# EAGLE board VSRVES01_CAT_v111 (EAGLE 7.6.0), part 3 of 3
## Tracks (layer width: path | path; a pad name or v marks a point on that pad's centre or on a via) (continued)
HP_LEFT  (via drill 0.4) (continued)
  Top 0.3: 3.3,41.7 4.2,42.6 4.2,45 6.2,47 6.4,47.2 HP-OUT.4 | R29.2 10.25,48.15
  Bottom 0.2: 7.4,48.2 HP-OUT.4
  Bottom 0.3: v10.2,48.2 7.4,48.2 HP-OUT.4
HP_MUTE  (via drill 0.4)
  Top 0.2: U4.4 3.2,40.4 5,38.6 v5,38.2 | v3.2,37.6 3.2,35.8 4,35 4.15,35 R37.1
  Bottom 0.2: v5,38.2 3.8,38.2 v3.2,37.6
HP_RIGHT
  Top 0.2: U4.13 9.1,41.7 9.2,41.8
  Top 0.3: 9.2,41.8 9.2,45 8.6,45.6 8.6,46.4 9.2,47 9.2,52.1 HP-OUT.1 9.9,52.75 R27.2
INT_N
  Top 0.2: U2.38 44.2,66.38 44.2,67 43.8,67.4 43.8,68 43.8,68.4 44,68.6 R7.1
LINE_ADC_L  (via drill 0.3)
  Top 0.2: U1.81 v17.4,39.02 | v8.6,55.4 6.6,55.4 5.8,56.2 R24.2 5.78,57.33 C25.1
  Bottom 0.2: v17.4,39.02 17.4,40.4 16.4,41.4 16.4,46.8 15.6,47.6 15.6,52.4 12.6,55.4 v8.6,55.4
LINE_ADC_R  (via drill 0.3)
  Top 0.2: U1.80 18,38.99 v18,39.49 | v11.4,56.2 11.2,56.4 R25.2 9.43,57.35 C27.1
  Bottom 0.2: v18,39.49 18,40.4 16.8,41.6 16.8,47 16,47.8 16,52.6 12.6,56 11.6,56 v11.4,56.2
MCT1  (via drill 0.4)
  Top 0.2: v35.8,67.2 C11.1
  Bottom 0.2: J1.P2 22.64,72.4 30,72.4 31,71.4 31,68.4 32.2,67.2 v35.8,67.2
MCT2  (via drill 0.4)
  Top 0.2: C10.1 v34.2,66.4
  Bottom 0.2: J1.P5 27.07,66.4 v34.2,66.4
MDC  (via drill 0.3)
  Top 0.2: U1.59 29.2,40.78 29.2,44.6 30.8,46.2 35.4,46.2 35.8,45.8 45.6,45.8 v46.4,46.6 | U2.36 46.4,66.09 46.4,67 47.2,67.8 v47.6,67.8 R9.1
  Bottom 0.2: v46.4,46.6 49.4,49.6 51.4,49.6 51.6,49.8 51.6,57.4 53.6,59.4 53.6,64.6 52.6,65.6 49.4,65.6 47.6,67.4 v47.6,67.8 47,67.8 46.6,67.4 45.6,67.4 45,68 45,75.4 44.13,76.27 JP3.2
MDIO  (via drill 0.3)
  Top 0.2: U1.58 29.6,40.61 29.6,44.4 31,45.8 35.2,45.8 35.8,45.2 46,45.2 v46.8,46 | U2.37 44.8,66.49 44.8,67.2 45.6,68 v45.8,68 R8.1
  Bottom 0.2: v46.8,46 50,49.2 51.8,49.2 52,49.4 52,57.2 54,59.2 54,65 53,66 49.6,66 48.2,67.4 48.2,68.2 47.8,68.6 46.6,68.6 46,68 v45.8,68 45.8,80.8 46.67,81.67 JP3.3
MX1+  (via drill 0.3)
  Top 0.2: U2.2 41.22,60.2 34.2,60.2 33.8,60.6 v33,60.6
  Bottom 0.2: J1.P1 19.95,67.25 22.2,65 30.6,65 33,62.6 v33,60.6
MX1-  (via drill 0.3)
  Top 0.2: U2.3 41.52,59.8 v33.6,59.8
  Bottom 0.2: J1.P3 22.5,66.91 23.8,65.6 31,65.6 33.6,63 v33.6,59.8
MX2+
  Top 0.2: U2.5 40.94,57.8 34.6,57.8 32,60.4 32,64.6 30.2,66.4 30.2,71.6 29.4,72.4 25.18,72.4 J1.P4
MX2-
  Top 0.2: U2.6 41.25,57.4 34.2,57.4 31.4,60.2 31.4,64.4 29.6,66.2 29.6,69 28.8,69.8 27.48,69.8 J1.P6
N$1
  Top 0.2: JMP1.1 14.95,44.8 14.31,44.8 14.01,44.5 U3.4 13.55,43.55 13.2,43.2 12,43.2 11.65,42.85 U3.1
N$2  (via drill 0.4)
  Top 0.2: U2.16 47.39,58.21 48,57.6 48,57 48.2,56.8 | 47.08,55.08 C33.1 | U2.40 43.4,65.77 43.4,66.2 43.14,66.46 41.8,66.46 41.6,66.66 41.6,67 | U2.34 48.92,67.2 | 46.08,55.08 v46.1,55.1
  Top 0.3: 48.2,56.8 48.2,56.2 47.08,55.08 | 48.92,67.2 50.2,67.2 v50.8,67.8 51,68 C16.1 | v46.4,56 46.4,55.6 46.8,55.2 46.88,55.2 C33.1 46.08,55.08 45.8,54.8 45.8,51.6 FB5.2 45.2,51.6 44.2,50.6 44.2,50.2 43.4,49.4 C43.1 | C17.1 41.6,67 v42.2,67
  POW 0.4: v42.2,67 48.4,67 | 48.4,67 48.6,67.2 50.2,67.2 v50.8,67.8 | 48.4,67 48.4,63.2 49.2,62.4 49.2,59.8 46.4,57 v46.4,56 46.4,55.4 v46.1,55.1
  Bottom 0.3: C114.1 v46.4,56 | C121.1 41.8,67 v42.2,67
N$3
  Top 0.2: U7.7 4.12,19.35 C66.2 4.67,18.07 4.4,17.8 1.8,17.8 0.6,19 0.6,25.6 0.95,25.95 R50.2 0.95,28.5 R43.1
N$4
  Top 0.2: C61.2 8.35,26.8 R44.1 | R41.2 6.65,26.82 C61.2 | U7.1 6,25 6.67,25.68 C61.2
N$5  (via drill 0.4)
  Top 0.2: 39.2,60.8 39.4,61.2 | 39.4,61.2 39.2,61.4 | U2.12 44.8,56.71 C32.1 | U2.1 40.91,60.6 40,60.6 39.8,60.8 39.4,60.8 39.4,61.2
  Top 0.3: C22.1 39.2,61.4 | 41.48,53 C37.1 | 44.73,55 C32.1
  Top 0.4: 39.2,61.4 v40,61.4 | FB4.2 39.8,52.8 41.48,52.8 41.48,53 | C37.1 C38.1 43.2,54.4 v43.8,55 44.73,55
  Bottom 0.3: C117.1 39.2,61.4 v40,61.4
  Bottom 0.4: v43.8,55 43.8,57.6 v40,61.4
N$6  (via drill 0.3)
  Top 0.2: RE.C 44.6,42.4 44.4,42.2 42.4,42.2 42.2,42.4 v41.2,42.4
  Bottom 0.2: v41.2,42.4 42.4,41.2 R3.2
N$7  (via drill 0.3)
  Top 0.2: LE.C v39.4,42.2
  Bottom 0.2: v39.4,42.2 40.2,41.4 R4.2
N$8  (via drill 0.4)
  Top 0.2: U2.9 41.57,55.6 | U2.4 41.03,58.6
  Top 0.3: 41.57,55.6 v40,55.6 C30.1
  Top 0.4: 41.03,58.6 v40,58.6 39.8,58.8 C24.1 | FB3.2 37.4,53 37.3,53 v37.3,54
  Bottom 0.3: C116.1 39.2,57.8 | C115.1 39.4,56.2 v40,55.6
  Bottom 0.4: 39.2,57.8 v40,58.6 | v37.3,54 38.4,54 38.5,54.1 39.08,54.67 C115.1 C116.1
N$9  (via drill 0.4)
  Top 0.2: U2.44 42.03,64.31 | 42.03,64.31 41.14,65.2 38.2,65.2 37.4,66 v37.4,67.8 | v37.4,67.8 37.4,68.2 | 37.4,68.2 C12.1 | 37.4,68.2 v37.4,67.8 | 42.03,64.31 42.03,64.57 v42,64.6 | v36.4,72.4 C9.1 37.2,72.53 FB2.2
  Bottom 0.2: v37.4,67.8 37.2,67.8 36.4,68.6 v36.4,72.4
  Bottom 0.3: C119.1 42.4,64.2 v42,64.6
N$11
  Top 0.2: U5.2 11.47,62.08 11.8,62.4 11.93,62.4 C21.1 | C21.1 14.07,62.67 14.2,62.8 13.95,62.8 R21.1 | R16.2 C21.1
N$12
  Top 0.2: R26.1 13.05,57.4 13.8,57.4 15,58.6 15,64 14.6,64.4 R16.1 13.85,65.75 13.4,66.2 XC2.+
N$13
  Top 0.2: R23.1 1.25,58.15 0.4,59 0.4,65.85 R14.1 4.6,70.05 4.6,75 12,82.4 XC1.+
N$14
  Top 0.2: R11.2 3.4,66.85 3.4,67.6 4.6,68.8 5.4,68.8 ADC_JACK.4 8.8,72.2 8.8,76.2 9.6,77 11,77 11.8,76.2 TV2.1 12.9,76.2 12.9,79.2 XC1.-
N$15  (via drill 0.4)
  Top 0.2: C35.1 50.27,55.08 C34.1 48.67,54.88 | U2.18 49.2,57.85 | 47.6,52 47.6,51.88 C39.1 | 47.33,48.52 FB6.2 | U2.39 43.8,66.08 43.8,66.4 | U2.30 49.55,65 | U2.26 50.58,63.2 v51,63.2 | U2.23 50.98,59.6
  Top 0.3: 49.2,57.85 49.2,56.8 49,56.6 C34.1 | 48.67,54.88 v48,54.2 48,52.4 47.6,52 | C39.1 C40.1 47.33,48.52 | 43.8,66.4 42.4,67.8 v42.4,68 42.2,68.2 C15.1 C14.1 C13.1 | 49.55,65 v50.6,65 53,67.4 C19.1 | 50.27,55.08 v49.8,55 | 50.98,59.6 51.52,59.06 53.14,59.06 53.26,59.26
  Top 0.4: v52.4,59.8 52.73,59.8 53.26,59.26 C23.1
  POW 0.4: v49.8,55 48.8,55 | 48.8,55 48.8,56.4 51.6,59.2 51.8,59.2 v52.4,59.8 | 48.8,55 v48,54.2
  Bottom 0.3: 49.67,64.47 C120.1 49.6,64.47 49.6,64.6
  Bottom 0.4: v52.4,59.8 51.8,60.4 51,60.4 49.67,61.73 C118.1 | 49.6,64.6 47.2,67 44.6,67 43.6,68 v42.4,68 | 49.8,64.4 C120.1 C118.1 | 49.6,64.47 49.88,64.47 50.4,65 v50.6,65 | C118.1 49.8,62.8 50.2,63.2 v51,63.2
N$16
  cutout GND: 20.92,84.58 20.92,82.08 26.92,82.08 26.92,84.58
  cutout POW: 20.92,84.58 20.92,82.08 26.92,82.08 26.92,84.58
N$17
  Top 0.2: PWR.C 58.6,1 58,0.4 56.05,0.4 R64.2
N$18
  Top 0.2: R12.2 R15.1
N$19  (via drill 0.3)
  Top 0.2: USD.12 58.95,32.55 v59,32.6
N$20
  Top 0.2: R5.2 10.25,69.85 11.6,71.2 XC2.- 12.9,71.2 12.9,73.6 TV1.1 11,73.6 10.1,74.5 ADC_JACK.1
N$21
  Bottom 0.2: R65.1 55,36.4 53.8,37.6 49.6,37.6 48.65,36.65 U11.4
N$22
  Bottom 0.2: Q1.1 53.15,23.6 C7.1 54.92,25.15 R65.2
N$23  (via drill 0.4)
  Top 0.2: C60.1 52.2,26.4
  Top 0.3: 53.7,27.85 53.85,27.85
  Top 0.4: USD.4 53.85,27.85 | 52.2,26.4 v52.2,27.3 | C60.1 53.7,27.85
  Bottom 0.2: R67.1 52.2,28.4 v52.2,27.3
  Bottom 0.4: Q1.3 v52.2,27.3
N$24  (via drill 0.3)
  Top 0.2: SDPW.A v53.2,33
  Bottom 0.2: R67.2 54,28.4 54,32.2 v53.2,33
N$27
  Top 0.2: R40.2 R41.1 4.92,28.38 C61.1 4.12,26 U7.2
N$30
  Top 0.2: U7.6 3.48,19.35 C66.1 1.8,18.8 1.2,19.4 1.2,25.4 2.6,26.8 R50.1 2.65,28.5 R52.2
N$45
  Top 0.2: R24.1 5.8,59.4 4.8,60.4 3,60.4 2.4,59.8 1.6,59.8 | 1.6,59.8 1.45,59.8 R23.2 | 1.6,59.8 1.6,61.35 | 1.6,61.35 R19.2 | 1.6,61.35 1.77,61.52 C20.2 2.92,61.6 2.8,61.6 3.6,61.6 4.08,62.08 U5.7
N$46
  Top 0.2: R25.1 R26.2 13.65,59.05 14,59.4 14,60.75 R21.2 12.22,60.95 C21.2 11.28,60.92 10.8,61.4 9.82,61.4 U5.1
N$48
  Top 0.2: 1.4,65.2 R14.2 R19.1 2.98,63.25 C20.1 3.12,63.4 3.6,63.4 4.28,62.73 U5.6
N$55
  Top 0.2: JP1.2 R63.2
N$75  (via drill 0.3)
  Top 0.2: RP4.6 52.4,48.8 51,50.2 v51,50.4 | U2.17 48.6,57.74 v48.6,57.4 | R1.2 18.8,57.6 19.2,57.2 24.4,57.2 25.6,58.4 25.6,59.4 26.8,60.6 29.4,60.6 33.8,56.2 34.8,56.2 35.2,55.8 35.2,55 35.6,54.6 41,54.6 41.4,54.2 v42.2,54.2
  Bottom 0.2: v51,50.4 49.8,51.6 49.8,53.4 48.6,54.6 v48.6,57.4 45.8,57.4 45.2,56.8 45.2,55.2 44.2,54.2 v42.2,54.2
N$77  (via drill 0.3)
  Top 0.2: RP4.4 52.6,48 v50.2,50.4 | U2.15 47.6,57.33 v47.6,56.6 | R2.2 24.35,58.55 24.8,59 24.8,60.2 25.8,61.2 29.6,61.2 v34,56.8
  Bottom 0.2: v50.2,50.4 48.2,52.4 47.6,52.4 | 47.6,52.4 46.8,51.6 43.2,51.6 42.4,52.4 36.8,52.4 34,55.2 v34,56.8 | v47.6,56.6 47.2,56.2 47.2,54 47.6,53.6 47.6,52.4
N$78  (via drill 0.3)
  Top 0.2: RP3.2 52,51.2 51.2,52 v50.8,52 | RP2.2 v53,55.2 | U2.19 49.6,58.15 v49.6,56.2
  POW 0.2: v53,55.2 50.6,55.2 v49.6,56.2
  Bottom 0.2: v50.8,52 50.8,55.2 50.2,55.8 50,55.8 v49.6,56.2
N$79  (via drill 0.3)
  Top 0.2: RP3.4 52.4,52 51.6,52.8 51.6,56 51.2,56.4 v50.4,56.4 50.4,56.6 50,57 50,58.46 U2.20 | RP2.4 v53,56
  POW 0.2: v53,56 50.8,56 v50.4,56.4
N$80  (via drill 0.3)
  Top 0.2: RP3.6 52.4,52.8 52,53.2 52,56.4 51.2,57.2 v50.8,57.2 50.4,57.6 50.4,58.77 U2.21 | RP2.6 v53,56.8
  POW 0.2: v53,56.8 51.2,56.8 v50.8,57.2
N$81  (via drill 0.3)
  Top 0.2: RP3.8 52.6,53.6 52.4,53.8 52.4,57 | 52.4,57 v51.4,58 51.2,58 50.8,58.4 50.8,59.08 U2.22 | RP2.8 53,57.6 52.4,57
N$82
  Top 0.2: U2.24 51.15,62 51.6,62 52.6,63 R20.2
  Top 0.3: R22.1 R20.2
N$83
  Top 0.2: U2.25 50.69,62.6 51.6,62.6 52.2,63.2 52.2,64.4 52.8,65 R17.1 53.4,65
N$84
  cutout Top: 15.4,40.2 18.2,40.2 18.2,40.4 15.4,40.4
N$93  (via drill 0.3)
  Top 0.2: RP4.8 52.4,49.6 51.6,50.4 51.6,50.6 v51,51.2 | U2.41 42.8,65.66 v42.67,65.94
  Bottom 0.2: v51,51.2 50.8,51.4 50.6,51.4 50.2,51.8 50.2,53.6 49,54.8 49,56.6 49.2,56.8 49.2,57.8 47.6,59.4 46.8,59.4 43.6,62.6 43.6,65.01 v42.67,65.94
N$95
  Top 0.2: U2.48 40.31,63.2 39,63.2 39,63.02 R18.1
  Top 0.3: R18.1 39.4,63
N$114
  Top 0.2: X1.4 50.6,8.2 50,8.8 R55.1
N$167
  Top 0.2: BUT1.P1 BUT1.P2 35.15,8.82 R56.1
N$168
  Top 0.2: R58.1 42.8,9.05 42.8,8.8 41.92,7.92 BUT2.P2 BUT2.P1
N$178
  Top 0.2: U4.5 1.35,39.75 1.2,39.6 1.2,37 1.8,36.4 2.12,36.4 C55.1
N$181
  Top 0.2: U4.14 8.3,43.77 C48.2
N$182
  Top 0.2: C47.2 3.08,42.88 2.6,42.4 2.15,42.4 U4.1
N$185
  Top 0.2: U4.12 10.3,41.05 R32.1
N$186  (via drill 0.4)
  Top 0.2: U4.9 7.3,39.1 v7,38.8 | v5.8,37.6 5.8,36.88 C54.1
  Bottom 0.2: v7,38.8 v5.8,37.6
N$187
  Top 0.2: U4.6 3.5,39.1 4.2,38.4 4.2,36.73 C54.2
N$202
  Top 0.2: U1.85 18.16,36 12.4,36 11.45,35.05 R36.1
N$203
  Top 0.2: U1.84 18.32,36.4 13.6,36.4 12.8,36.4 12.2,37 R35.1
NLL
  Top 0.2: J1.L2 25.11,61.4 21.8,61.4 21.4,61 R2.1
NLR
  Top 0.2: J1.L4 18.93,60.25 R1.1
OP_AMP_BUFFER  (via drill 0.4)
  Top 0.2: v14.8,67 15.4,66.4 15.4,57.6 12.8,55 12.8,48.8 16.2,45.6 16.2,43.6 15.75,43.15 JMP1.2 | 10,67 R13.1 v11.2,67
  Bottom 0.2: v14.8,67 v11.2,67
Q1N1
  Top 0.2: U2.45 42.4,63.2 40.8,64.8 33.8,64.8 32.8,66 32.8,71.2 35.8,74.2 35.8,75 36.2,75.4 40.4,75.4 43.2,72.6 46.6,72.6 47.8,73.8 47.8,76.2 47,77 46.45,77 XTAL1.3 46.35,78.53 C3.1 C2.1
Q1P1
  Top 0.2: U2.46 40.52,64.4 33.6,64.4 32.4,65.8 32.4,71.4 35.4,74.4 35.4,75.2 36,75.8 41.12,75.8 41.6,75.33 C6.1 42.48,75.4 42.8,75.4 42.9,75.3 XTAL1.1 44.33,75.03 C8.1
RCAP
  Top 0.2: U3.3 13.96,41.9 14.41,41.45 JMP1.3 15,40.6 14.53,40.12 C52.1 14.53,38.67 14.8,38.4 17.45,38.4 U1.82
RX_CTL
  Top 0.2: U1.57 30,40.45 30,44.2 30.4,44.6 32.55,44.6 R30.2
RX_CTL_RES  (via drill 0.3)
  Top 0.2: R30.1 46.8,44.8 47.6,45.6 v47.6,46 | U2.33 49.03,66.6 v49.8,66.6
  Bottom 0.2: v47.6,46 47.6,46.2 50.2,48.8 52.2,48.8 52.4,49 52.4,57 54.4,59 54.4,65.4 53.2,66.6 v49.8,66.6
RX_RV
  Top 0.2: U1.43 30.97,32.8 31.4,32.8 36.2,28 36.2,13.2 28.6,5.6 26.6,5.6 24,3 20.8,3 19,4.8 19,5.6 11.8,12.8 R53.1 10.4,12.85 10.4,13.6 10.14,13.86 UART_RV.P$2
RX_VSDSP  (via drill 0.3)
  Top 0.2: U1.68 23.2,40.57 23.2,41 24.4,42.2 24.4,45.6 27.4,48.6 27.4,49.2 28.2,50 28.4,50 v28.8,49.6 | v38.2,35.6 39,35.6 39.2,35.8 50,35.8 51.05,36.85 R34.1 51.05,39.25 52.86,41.06 UART_VSDSP.P$2
  Bottom 0.2: v28.8,49.6 29.8,49.6 36.2,43.2 36.2,38.2 38.2,36.2 v38.2,35.6
RXC_D  (via drill 0.3)
  Top 0.2: U1.51 31.55,38.6 44.6,38.6 51,45 51,46.2 v51.4,46.6 | v57.8,56.8 58.4,57.4 58.4,71.4 57.2,72.6 54.6,72.6 54.4,72.4 53.2,72.4 52.2,71.4 49.8,71.4 49.4,71 R10.2
  Bottom 0.2: v51.4,46.6 54,46.6 54.4,47 54.4,52.6 55.2,53.4 55.2,54.2 v57.8,56.8
RXC_RES  (via drill 0.3, 0.4)
  Top 0.2: U2.35 48.82,67.8 v49.4,67.8 R10.1 | R6.2 49.2,72.4 v48.4,71.6
  Bottom 0.2: v49.4,67.8 49.4,70.6 v48.4,71.6
RXD0-M0
  Top 0.2: U1.52 31.78,39.4 RP5.2
RXD0-M0_RES  (via drill 0.3)
  Top 0.2: RP5.1 44.8,39.4 50.4,45 v50.4,46.4 | U2.32 49.14,66 50,66 52,68 52,69.6 53.6,71.2 RP1.8 | RP1.8 54.4,71.4 | RP1.8 54.4,71.8 54.8,72.2 56.8,72.2 57.8,71.2 v57.8,58.2
  Bottom 0.2: v50.4,46.4 50.4,46.6 51,47.2 53.8,47.2 54,47.4 54,52.8 54.8,53.6 54.8,54.4 57,56.6 57,57.4 v57.8,58.2
RXD1-M1
  Top 0.2: U1.53 32.01,40.2 RP5.4
RXD1-M1_RES  (via drill 0.3)
  Top 0.2: RP5.3 45,40.2 49.8,45 v49.8,45.4 | U2.31 49.45,65.6 50.2,65.6 52.4,67.8 52.4,69.4 53.4,70.4 v53.6,70.4 RP1.6
  Bottom 0.2: v49.8,45.4 49.8,46.6 50.8,47.6 53.4,47.6 53.6,47.8 53.6,53 54.4,53.8 54.4,54.6 56.4,56.6 56.4,62.4 58,64 58,65.8 58,66.8 56.2,68.6 56.2,69.2 55,70.4 v53.6,70.4
RXD2-M2
  Top 0.2: U1.54 31.2,39.95 31.2,40.6 31.6,41 31.8,41 RP5.6
RXD2-M2_RES  (via drill 0.3)
  Top 0.2: RP5.5 45.2,41 49,44.8 v49,45.4 | U2.28 50.17,64.2 50.6,64.2 52.8,66.4 56.2,66.4 56.4,66.6 v57.2,66.6 | RP1.4 v53.6,69.6
  Bottom 0.2: v49,45.4 49,46.4 50.6,48 52.8,48 53.2,48.4 53.2,53.2 54,54 54,54.8 56,56.8 56,58.6 55.2,59.4 55.2,63.6 57.2,65.6 v57.2,66.6 55.8,66.6 55.4,67 55.4,69 54.8,69.6 v53.6,69.6
RXD3-M3
  Top 0.2: U1.55 30.8,40.12 30.8,41 31.6,41.8 RP5.8
RXD3-M3_RES  (via drill 0.3)
  Top 0.2: RP5.7 38,41.8 38.2,41.6 45,41.6 48.2,44.8 v48.2,45.6 | U2.27 50.48,63.8 50.8,63.8 53,66 v56.6,66 | RP1.2 v53.6,68.8
  Bottom 0.2: v48.2,45.6 48.2,46.2 50.4,48.4 52.4,48.4 52.8,48.8 52.8,54.2 54.4,55.8 54.4,58.4 54.8,58.8 54.8,66 | v53.6,68.8 RP1.2 54.8,68.4 54.8,66 | 54.8,66 v56.6,66
TX_CTL  (via drill 0.3)
  Top 0.2: U1.50 31.71,38.2 44.8,38.2 51.8,45.2 v51.8,45.8 | v58.8,54.8 58.8,55 57.2,56.6 57.2,60.8 56.8,61.2 56.8,64.4 56.2,65 R17.2
  Bottom 0.2: v51.8,45.8 53.8,45.8 54.8,46.8 54.8,52.4 55.8,53.4 55.8,54 56,54.2 58.2,54.2 v58.8,54.8
TX_RV
  Top 0.2: U1.44 31.37,33.43 36.6,28.2 36.6,13 29,5.4 29,3.8 28.4,3.2 26,3.2 25.4,2.6 20.6,2.6 18.4,4.8 18.4,5.6 14.4,9.6 R54.1 10.45,10.95 10.08,11.32 UART_RV.P$3
TX_VSDSP  (via drill 0.3)
  Top 0.2: U1.67 24.8,41.47 24.8,45.4 28,48.6 28,48.8 v28.2,49 | R33.1 v37.6,35 39,35 39.4,35.4 51.6,35.4 54.72,38.52 UART_VSDSP.P$3
  Bottom 0.2: v28.2,49 29.8,49 35.6,43.2 35.6,38 37.4,36.2 37.4,35.2 v37.6,35
TXC
  Top 0.2: U1.45 32.54,36.2 45.8,36.2 54.4,44.8 57.4,44.8 59.2,46.6 59.2,53.4 56.8,55.8 56.8,60 56,61 R22.2
TXD0  (via drill 0.3)
  Top 0.2: U1.46 32.37,36.6 35.8,36.6 38.8,36.6 45.6,36.6 54.2,45.2 57.2,45.2 58.8,46.8 58.8,50.8 v58.4,51.2 | RP3.1 v55.8,51.2
  Bottom 0.2: v58.4,51.2 v55.8,51.2
TXD1  (via drill 0.3)
  Top 0.2: U1.47 32.21,37 35.8,37 39,37 45.4,37 54,45.6 57,45.6 58,46.6 58.2,46.8 v58.2,50.2 | RP3.3 v56,52
  Bottom 0.2: v58.2,50.2 58.6,50.2 59.2,50.8 59.2,51.8 58.8,52.2 56.2,52.2 v56,52
TXD2  (via drill 0.3)
  Top 0.2: U1.48 32.04,37.4 45.2,37.4 53.8,46 56.6,46 57.6,47 57.6,51.6 58.2,52.2 v58.2,53.2 | RP3.5 v56.2,52.8
  Bottom 0.2: v58.2,53.2 56.6,53.2 v56.2,52.8
TXD3
  Top 0.2: U1.49 31.88,37.8 35.8,37.8 39.4,37.8 45,37.8 53.6,46.4 56.2,46.4 57,47.2 57,53.2 56.6,53.6 RP3.7
USB_RV+  (via drill 0.3)
  Top 0.2: U1.87 17.83,35.2 17.4,35.2 16.2,34 15,34 11.4,30.4 11.4,23.4 10.6,22.6 10.2,22.6 v9.8,22.2 | v49.2,5 49.2,6.8 49.8,7.4 X1.3
  Bottom 0.2: v9.8,22.2 7.8,20.2 7.8,12.6 11.8,8.6 14.6,8.6 15.8,7.4 15.8,4.8 19.2,1.4 25.6,1.4 26.4,0.6 28.2,0.6 30.4,2.8 46.8,2.8 49,5 v49.2,5
USB_RV-  (via drill 0.3)
  Top 0.2: U1.88 17.57,34.57 16.6,33.6 15.2,33.6 11.8,30.2 11.8,23.2 v10.2,21.6 | X1.2 50,6.6 v49.8,6.4
  Bottom 0.2: v10.2,21.6 9.8,21.2 9.4,21.2 8.2,20 8.2,12.8 12,9 14.8,9 16.2,7.6 16.2,5 19.4,1.8 25.8,1.8 27.2,3.2 46.6,3.2 v49.8,6.4
VREFA  (via drill 0.2)
  Top 0.11: v13.2,15 12.88,15.32 C69.1 12.72,15.4
  Top 0.2: R51.2 12.72,15.4
  Top 0.3: R49.1 R51.2
  Bottom 0.1: 20.09,15.2 19.74,14.84
  Bottom 0.11: U100.G3 20.7,15.5 20.4,15.2 20.09,15.2 | 19.74,14.84 13.47,14.84 v13.2,15
VREFQ  (via drill 0.2)
  Top 0.2: C76.1 20.73,8.28 v20.6,8.6
  Top 0.3: C76.1 21.12,6.22 R59.2 R60.1
  Bottom 0.2: U100.J9 22,10 v20.6,8.6
XCKB  (via drill 0.2)
  Top 0.11: v31.2,32.2 arc65 30.9,32.4 arc-25 30.64,32.56 U1.42
  Bottom 0.11: U100.H3 21.32,15.66 21.4,15.66 21.68,15.93 21.68,17.34 21.68,17.55 21.4,18 21.4,19.75 21.4,20.6 | v31.2,32.2 arc-90 30.8,31.6 30.4,31.2 30.4,31 29.6,30.2 29.6,30 29.6,23.6 29.6,23 28.8,22.2 28.3,22.2 arc-90 28.12,22.38 28.12,22.42 arc90 27.95,22.59 27.84,22.59 arc90 27.66,22.42 27.66,21.98 arc-90 27.49,21.81 27.38,21.81 arc-90 27.2,21.98 27.2,22.42 arc90 27.03,22.59 26.92,22.59 arc90 26.74,22.42 26.74,21.98 arc-90 26.57,21.81 26.46,21.81 arc-90 26.28,21.98 26.28,22.42 arc90 26.11,22.59 26,22.59 arc90 25.82,22.42 25.82,21.98 arc-90 25.64,21.81 25.53,21.81 arc-90 25.36,21.98 25.36,22.42 arc90 25.18,22.59 25.07,22.59 arc90 24.9,22.42 24.9,21.98 arc-90 24.72,21.81 24.61,21.81 arc-90 24.44,21.98 24.44,22.42 arc90 24.26,22.59 24.15,22.59 arc90 23.98,22.42 23.98,22.38 arc-90 23.8,22.2 22.8,22.2 22.6,22.2 22,21.6 21.4,21 21.4,20.6 | R100.2 21.4,20.6
XRST_ETH  (via drill 0.3)
  Top 0.2: U2.42 41.75,66 v38.2,66 | U1.76 19.8,39.45 19.8,41.05 18.55,42.3 R31.1 18.6,43.45 v18.6,44.4 C44.1 | v35.8,35.4 35.8,29.6 37,28.4 37,12.8 29.4,5.2 29.4,1.8 28.2,0.6 27,0.6 25.8,1.8 RESET.S1 RESET.S2
  Bottom 0.2: v18.6,44.4 20,44.4 20.6,43.6 28.8,43.6 | 28.8,43.6 32.4,43.6 34.2,41.8 34.2,37.6 35.8,36 v35.8,35.4 | 28.8,43.6 28.8,45.6 26.6,47.8 26.6,53 25.6,54 25.6,55.6 26.6,56.6 31.6,56.6 34.6,59.6 34.6,61.4 38.2,65 v38.2,66
XTALI_UI
  Top 0.2: U1.77 19.4,39.28 19.4,40.68 17.6,42.48 17.6,47.8 19.05,49.25 R28.2 C42.2 20.73,52.17 XTAL2.2 19.52,54.23 C29.2
XTALO_UI
  Top 0.2: U1.78 19,39.12 19,40.32 17.2,42.12 17.2,48 17.55,48.35 R28.1 17.4,49.6 | 17.6,49.4 17.4,49.6 | 17.4,49.6 C41.2 16.07,52.17 XTAL2.1 17.27,54.23 C28.2
ZQ1  (via drill 0.2, 0.3)
  Top 0.3: R48.2 v11.8,19.2
  POW 0.3: v15.2,16.4 15.2,18.2 14.2,19.2 v11.8,19.2
  Bottom 0.11: U100.D3 18.72,15.66 18.54,15.66 18.25,15.95 15.65,15.95 v15.2,16.4

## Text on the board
Top: 1
GND: 2
POW: 3
Bottom: 4
tPlace: ADC / JACK | VSRVES01 | +5V | RX | CAT | TX | GND | GND | C66 | v.1.1 / PL, Ski 4/2025 | 5V | R53 | RX | TX | GND
bPlace: R14 | R11 | R13 | C18 | R12 | R15 | R19 | C20 | C25 | R24 | C26 | C27 | Boxed components / are on top side | C47 | C48
tNames: C66 | GP1 / / GP0 / / GND
bNames: U2
tDocu: GND
_tNames: R13 | R14 | R12 | R15 | C18 | R19 | C20 | C25 | R24 | C26 | C27 | C47 | C48 | R43 | R52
